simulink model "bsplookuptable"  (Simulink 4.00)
settings: Solver=ode45  StartTime=0.0  StopTime=20.0  RelTol=1e-3
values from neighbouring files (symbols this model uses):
  vecin = [-10:2:10]    [bsplookuptable_sim.m]
  vecout = [-5 -5 -5 -2 -2 -2 4.5 4.5 4.5 0 -1]    [bsplookuptable_sim.m]
libraries: simulink3 x1

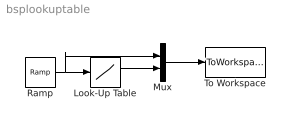
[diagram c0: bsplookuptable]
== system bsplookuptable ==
  Look-Up Table : Lookup  InputValues=vecin  OutputValues=vecout
  Mux : Mux  Inputs=2
  Ramp : simulink3/Sources/Ramp  slope=1  start=0  X0=-10
  To Workspace : ToWorkspace  VariableName=auslese  SampleTime=-1  SaveFormat=Array
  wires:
  Look-Up Table/1 -> Mux/2
  Ramp/1 -> Look-Up Table/1, Mux/1
  Mux/1 -> To Workspace/1
